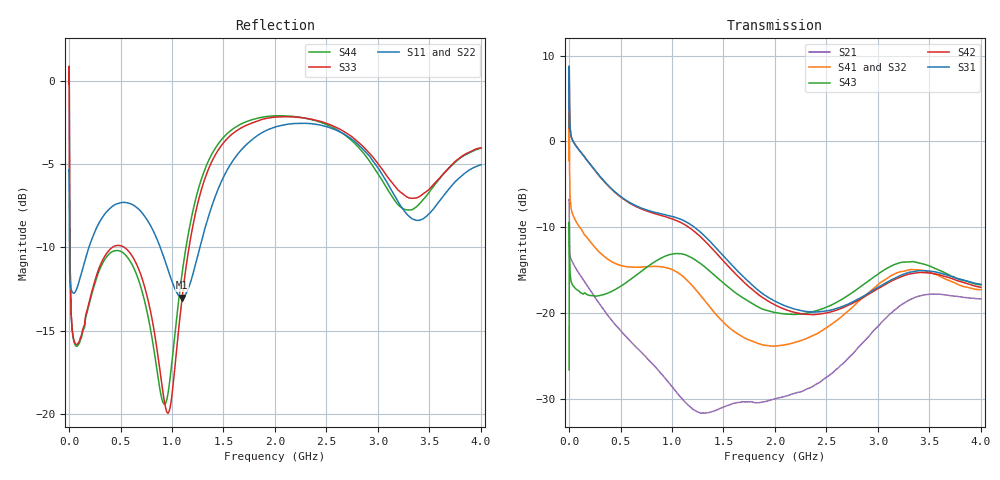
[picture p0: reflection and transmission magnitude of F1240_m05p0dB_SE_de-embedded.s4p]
! Integrated Device Technology
! Corporate Headquarters
! 6024 Silver Creek Valley Road
! San Jose, CA 95138  USA
! Phone:  1-408-284-8200
! Toll Free:  1-800-223-1366
! Webpage:  http://www.idt.com/
! Timing and RF Division
! 515 Groton Road, Suite 102
! Westford, MA 01886-6024
! Device:  F1240
! Description: Dual Intermediate Frequency Digital Variable Gain Amplifier
! Frequency:  10.0 -  500.00 MHz
! Package:  5x5 mm QFN Plastic Package: 32 pin
! Ports:  8 RF, 20 DC
!  Pin  1  = GA3 / Data  Pin 17  = RF OUT_B+
!  Pin  2  = GA4 / CLK  Pin 18  = RF OUT_B-
!  Pin  3  = GA5  Pin 19  = STBY_B
!  Pin  4  = VMODE  Pin 20  = Ground
!  Pin  5  = No Connect  Pin 21  = Ground
!  Pin  6  = GB5  Pin 22  = STB_A
!  Pin  7  = GB4  Pin 23  = RF OUT_A-  = Port 4
!  Pin  8  = GB3  Pin 24  = RF OUT_A+  = Port 3
!  Pin  9  = GB2  Pin 25  = GA0
!  Pin 10  = GB1  Pin 26  = ISET_A
!  Pin 11  = RF IN_B+  Pin 27  = VCC
!  Pin 12  = RF IN_B-  Pin 28  = Ground
!  Pin 13  = Ground  Pin 29  = RF IN_A-  = Port 2
!  Pin 14  = VCC  Pin 30  = RF IN_A+  = Port 1
!  Pin 15  = ISET_B  Pin 31  = GA1
!  Pin 16  = GB0  Pin 32  = GA2 / CSb
! Gain  = +19.5 dB
! State  = 1
! Voltage  = +5.00 V
! Current  = 85.292 mA (one channel only)
! Temperture  =  +25 C
! Test Date  =  2017-10-18
! Board  =  EB4031
! Data:  The device was measured on a custom evaluation board which has
!  individual transmission lines to the RF pins.  Data was collected
!  using a calibrated network analyzer.  The evaluation board was
!  de-embedded using Automatic Fixture Removal.
!  The reference plane is the edge of the package pin.
!  Only Channel A was measured.
!  This data is in single-ended operation.  If your needs are balanced
!  or differential S-parameters then this file needs to be used a
!  linear simulator.
! File Date:  2017-11-10  MJV
! Note:
!  Integrated Device Technology supplies this data as a sample of measured
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# Hz S dB R 100
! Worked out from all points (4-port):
!   410 points, 500 kHz to 4 GHz, reference 100 ohm
!   strongest paths, dB at 500 kHz, 930 MHz, 1.96 GHz, 2.98 GHz, 4 GHz:
!     S31: 1.6, -8.5, -18.4, -17.1, -16.7
!     S42: 1.6, -8.8, -18.8, -17.3, -17.0
!     S43: -26.6, -13.4, -19.8, -15.7, -16.7
!     S41: -2.2, -14.7, -23.9, -16.9, -17.3
!     S32: -2.2, -14.9, -23.8, -17.3, -17.7
!     S21: -6.8, -27.6, -30.1, -21.8, -18.4
!   lowest |S11| = -13.0 dB at 1.1 GHz (marker M1), VSWR 1.58, Z = 64.8 - j11.2 ohm
!   |S11| at or under -10 dB: 3.088 MHz to 192.6 MHz (189.5 MHz wide, 194 % of centre); 886 MHz to 1.27 GHz (384 MHz wide, 35.6 % of centre)
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500000  -5.40 -5.6  -6.82 -5.9  -31.06 79.0  -35.14 77.4
        -6.82 -5.9  -5.39 -5.6  -35.11 76.5  -31.05 80.1
        1.62 -109.5  -2.21 -111.6  -0.20 0.3  -26.64 -39.2
        -2.24 -110.5  1.62 -108.4  -26.63 -39.3  -0.20 2.6
2000000  -7.80 -31.4  -9.67 -32.1  -22.34 24.4  -27.13 6.0
         -9.67 -32.1  -7.78 -31.5  -27.09 5.8  -22.33 24.8
         8.22 179.3  3.76 162.8  -0.28 -51.7  -9.41 -141.2
         3.72 163.1  8.23 179.6  -9.41 -141.3  -0.32 -51.3
4000000  -10.89 -26.6  -12.67 -22.0  -22.90 6.7  -30.28 -13.5
         -12.67 -22.0  -10.89 -26.8  -30.24 -13.7  -22.90 6.9
         4.85 158.0  -1.95 139.7  -4.78 -84.1  -11.90 175.9
         -1.99 139.8  4.86 158.2  -11.89 175.8  -4.83 -84.1
3.9e8  -7.70 -136.8  -20.47 -104.9  -27.02 -83.1  -36.38 -67.2
       -20.48 -104.8  -7.60 -137.9  -36.50 -65.8  -27.18 -83.5
       -5.25 56.6  -13.91 12.6  -10.16 -161.7  -17.67 44.8
       -13.85 11.9  -5.31 55.4  -17.62 44.5  -10.38 -162.3
1.1e9  -13.01 -158.4  -30.34 153.6  -26.20 139.1  -33.20 178.0
       -30.04 152.8  -12.99 -156.8  -33.21 -177.4  -27.13 138.8
       -9.16 -107.5  -15.88 163.2  -12.92 -105.9  -13.29 -146.3
       -15.67 158.3  -9.55 -109.9  -13.12 -146.2  -11.46 -106.7
2.85e9  -4.07 106.1  -23.54 -24.2  -27.39 -150.8  -29.62 -135.4
        -23.51 -24.3  -3.85 106.7  -30.31 -122.8  -28.71 -144.6
        -18.12 -64.4  -18.62 -146.6  -3.90 103.4  -17.57 -80.6
        -18.27 -157.6  -18.25 -61.2  -16.78 -78.3  -4.26 96.6
4e9  -5.03 -131.0  -18.37 113.4  -26.08 -36.6  -27.09 -21.1
     -18.37 113.3  -4.74 -129.7  -27.77 -6.2  -27.93 -28.5
     -16.66 44.7  -17.72 -55.4  -4.01 -133.6  -18.20 63.8
     -17.28 -69.4  -17.02 50.6  -16.73 56.4  -4.05 -143.4
